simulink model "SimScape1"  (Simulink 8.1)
settings: Solver=ode45  StartTime=0.0  StopTime=.25  RelTol=1e-10
libraries: fl_lib x30, nesl_utility x6

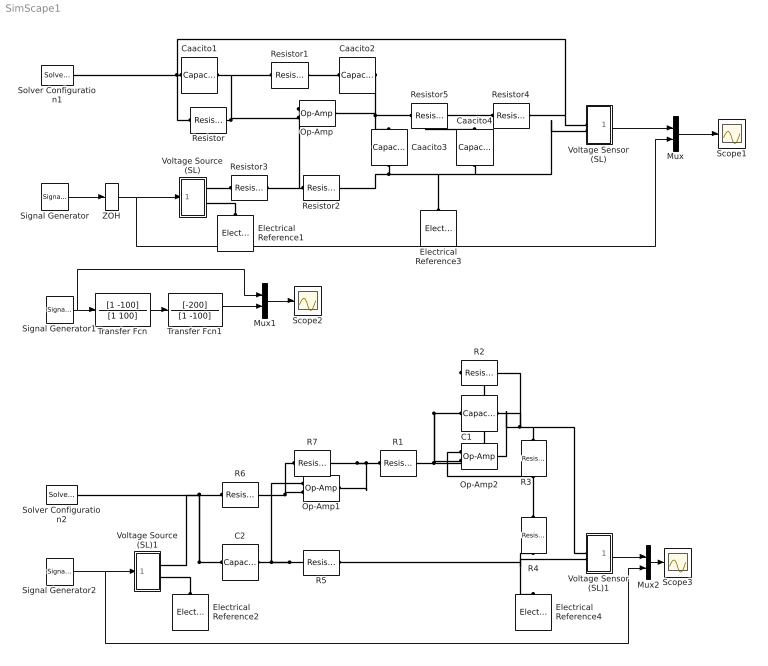
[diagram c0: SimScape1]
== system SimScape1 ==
  C1 : fl_lib/Electrical/Electrical Elements/Capacitor  c=2e-6 F  v0=0 V  r=1e-6 Ohm  g=0 1/Ohm  i_Log=off  v_Log=off  vc_Log=off  LocalVarNames=|i|v|vc  LocalVarDescs=|i|v|Internal variable for voltage across capacitor term  LocalVarLogging=[0 0 0]
  C2 : fl_lib/Electrical/Electrical Elements/Capacitor  c=1e-6 F  v0=0 V  r=1e-6 Ohm  g=0 1/Ohm  i_Log=off  v_Log=off  vc_Log=off  LocalVarNames=|i|v|vc  LocalVarDescs=|i|v|Internal variable for voltage across capacitor term  LocalVarLogging=[0 0 0]
  Caacito1 : fl_lib/Electrical/Electrical Elements/Capacitor  c=1e-6 F  v0=0 V  r=1e-6 Ohm  g=0 1/Ohm  i_Log=off  v_Log=off  vc_Log=off  LocalVarNames=|i|v|vc  LocalVarDescs=|i|v|Internal variable for voltage across capacitor term  LocalVarLogging=[0 0 0]
  Caacito2 : fl_lib/Electrical/Electrical Elements/Capacitor  c=1e-6 F  v0=0 V  r=1e-6 Ohm  g=0 1/Ohm  i_Log=off  v_Log=off  vc_Log=off  LocalVarNames=|i|v|vc  LocalVarDescs=|i|v|Internal variable for voltage across capacitor term  LocalVarLogging=[0 0 0]
  Caacito3 : fl_lib/Electrical/Electrical Elements/Capacitor  c=100e-6 F  v0=0 V  r=1e-6 Ohm  g=0 1/Ohm  i_Log=off  v_Log=off  vc_Log=off  LocalVarNames=|i|v|vc  LocalVarDescs=|i|v|Internal variable for voltage across capacitor term  LocalVarLogging=[0 0 0]
  Caacito4 : fl_lib/Electrical/Electrical Elements/Capacitor  c=100e-6 F  v0=0 V  r=1e-6 Ohm  g=0 1/Ohm  i_Log=off  v_Log=off  vc_Log=off  LocalVarNames=|i|v|vc  LocalVarDescs=|i|v|Internal variable for voltage across capacitor term  LocalVarLogging=[0 0 0]
  Electrical Reference{1..4} (4 alike) : fl_lib/Electrical/Electrical Elements/Electrical Reference  i_Log=off  LocalVarNames=|v1  LocalVarDescs=|v1  LocalVarLogging=[]
  Mux : Mux  Inputs=2
  Mux1 : Mux  Inputs=2
  Mux2 : Mux  Inputs=2
  Op-Amp : fl_lib/Electrical/Electrical Elements/Op-Amp  i1_Log=off  v1_Log=off  outI_Log=off  LocalVarNames=|i1|v1|outI  LocalVarDescs=|i1|v1|outI  LocalVarLogging=[0 0 0]
  Op-Amp1 : fl_lib/Electrical/Electrical Elements/Op-Amp  i1_Log=off  v1_Log=off  outI_Log=off  LocalVarNames=|i1|v1|outI  LocalVarDescs=|i1|v1|outI  LocalVarLogging=[0 0 0]
  Op-Amp2 : fl_lib/Electrical/Electrical Elements/Op-Amp  i1_Log=off  v1_Log=off  outI_Log=off  LocalVarNames=|i1|v1|outI  LocalVarDescs=|i1|v1|outI  LocalVarLogging=[0 0 0]
  R{1..3,5..7} (6 alike) : fl_lib/Electrical/Electrical Elements/Resistor  R=10 kOhm  i_Log=off  v_Log=off  LocalVarNames=|i|v  LocalVarDescs=|i|v  LocalVarLogging=[0 0]
  R4 : fl_lib/Electrical/Electrical Elements/Resistor  R=30 kOhm  i_Log=off  v_Log=off  LocalVarNames=|i|v  LocalVarDescs=|i|v  LocalVarLogging=[0 0]
  Resistor{,1..3} (4 alike) : fl_lib/Electrical/Electrical Elements/Resistor  R=1 kOhm  i_Log=off  v_Log=off  LocalVarNames=|i|v  LocalVarDescs=|i|v  LocalVarLogging=[0 0]
  Resistor4 : fl_lib/Electrical/Electrical Elements/Resistor  R=10 kOhm  i_Log=off  v_Log=off  LocalVarNames=|i|v  LocalVarDescs=|i|v  LocalVarLogging=[0 0]
  Resistor5 : fl_lib/Electrical/Electrical Elements/Resistor  R=10 kOhm  i_Log=off  v_Log=off  LocalVarNames=|i|v  LocalVarDescs=|i|v  LocalVarLogging=[0 0]
  Scope1 : Scope
  Scope2 : Scope
  Scope3 : Scope
  Signal Generator : SignalGenerator  WaveForm=square  Frequency=100
  Signal Generator1 : SignalGenerator  WaveForm=square  Frequency=10
  Signal Generator2 : SignalGenerator  WaveForm=square  Frequency=10
  Solver Configuration1 : nesl_utility/Solver Configuration  PhysicalDomain=network_engine_domain  SubClassName=solver  LeftPortType=input  RightPortType=generic  Accelerate=off  Tones=[]  Harmonics=[]  SimulateNoise=off  Profile=off  UseLocalSampling=off  EnableSwitchedLinearOptims=on  FrequencyDomain=off  UseCCode=off  UseNewInitialization=off  DoDC=off  ResidualTolerance=1e-4  UseLocalSolver=on  LocalSolverChoice=NE_BACKWARD_EULER_ADVANCER  LocalSolverSampleTime=.001  DoFixedCost=on  MaxNonlinIter=3  MaxModeIter=2  LinearAlgebra=Sparse  DelaysMemoryBudget=1024
  Solver Configuration2 : nesl_utility/Solver Configuration  PhysicalDomain=network_engine_domain  SubClassName=solver  LeftPortType=input  RightPortType=generic  Accelerate=off  Tones=[]  Harmonics=[]  SimulateNoise=off  Profile=off  UseLocalSampling=off  EnableSwitchedLinearOptims=on  FrequencyDomain=off  UseCCode=off  UseNewInitialization=off  DoDC=off  ResidualTolerance=1e-4  UseLocalSolver=on  LocalSolverChoice=NE_BACKWARD_EULER_ADVANCER  LocalSolverSampleTime=.001  DoFixedCost=on  MaxNonlinIter=3  MaxModeIter=2  LinearAlgebra=Sparse  DelaysMemoryBudget=1024
  Transfer Fcn : TransferFcn  Numerator=[1 -100]  Denominator=[1 100]
  Transfer Fcn1 : TransferFcn  Numerator=[-200]  Denominator=[1 -100]
  Voltage Sensor (SL) : Subsystem
  Voltage Sensor (SL)1 : Subsystem
  Voltage Source (SL) : Subsystem
  Voltage Source (SL)1 : Subsystem
  ZOH : ZeroOrderHold  SampleTime=.001
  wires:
  Signal Generator/1 -> ZOH/1
  Mux/1 -> Scope1/1
  Voltage Sensor (SL)/1(v) -> Mux/1
  ZOH/1 -> Voltage Source (SL)/1(S), Mux/2
  Signal Generator1/1 -> Transfer Fcn/1, Mux1/1
  Transfer Fcn/1 -> Transfer Fcn1/1
  Mux1/1 -> Scope2/1
  Transfer Fcn1/1 -> Mux1/2
  Signal Generator2/1 -> Voltage Source (SL)1/1(S), Mux2/2
  Mux2/1 -> Scope3/1
  Voltage Sensor (SL)1/1(v) -> Mux2/1
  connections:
  Caacito1/RConn1 -- Resistor/RConn1 -- Op-Amp/LConn2 -- Resistor1/LConn1
  Caacito1/LConn1 -- Resistor/LConn1 -- Resistor4/LConn1 -- Voltage Sensor (SL)/LConn1 -- Solver Configuration1/RConn1
  Resistor2/LConn1 -- Op-Amp/LConn1 -- Resistor3/LConn1
  Caacito2/LConn1 -- Resistor1/RConn1
  Caacito2/RConn1 -- Op-Amp/RConn1 -- Resistor5/RConn1 -- Caacito3/LConn1
  Resistor5/LConn1 -- Resistor4/RConn1 -- Caacito4/LConn1
  Caacito3/RConn1 -- Electrical Reference3/LConn1 -- Caacito4/RConn1 -- Voltage Sensor (SL)/LConn2 -- Resistor2/RConn1
  Electrical Reference1/LConn1 -- Voltage Source (SL)/RConn2
  Voltage Source (SL)/RConn1 -- Resistor3/RConn1
  R7/LConn1 -- R6/RConn1 -- Op-Amp1/LConn2
  C2/RConn1 -- Op-Amp1/LConn1 -- R5/LConn1
  R2/RConn1 -- C1/LConn1 -- Op-Amp2/LConn2 -- R1/RConn1
  R5/RConn1 -- R4/LConn1 -- Electrical Reference4/LConn1 -- Voltage Sensor (SL)1/LConn2
  Voltage Source (SL)1/RConn1 -- C2/LConn1 -- R6/LConn1 -- Solver Configuration2/RConn1
  Electrical Reference2/LConn1 -- Voltage Source (SL)1/RConn2
  R1/LConn1 -- R7/RConn1 -- Op-Amp1/RConn1
  R3/RConn1 -- C1/RConn1 -- Op-Amp2/RConn1 -- R2/LConn1 -- Voltage Sensor (SL)1/LConn1
  R3/LConn1 -- R4/RConn1 -- Op-Amp2/LConn1

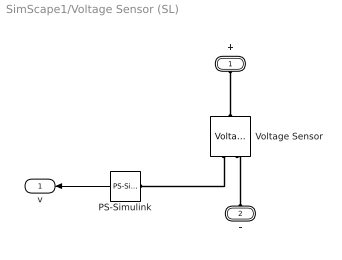
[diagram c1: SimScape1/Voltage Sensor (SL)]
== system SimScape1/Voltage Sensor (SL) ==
  PS-Simulink : nesl_utility/PS-Simulink Converter  PhysicalDomain=network_engine_domain  SubClassName=ps_output  LeftPortType=input  RightPortType=output  PseudoPeriodic=off  Frequencies=[]  Unit=V  AffineConversion=off
  Voltage Sensor : fl_lib/Electrical/Electrical Sensors/Voltage Sensor  i1_Log=off  v1_Log=off  LocalVarNames=|i1|v1  LocalVarDescs=|i1|v1  LocalVarLogging=[]
  + : PMIOPort  Port=1  Side=Left
  - : PMIOPort  Port=2  Side=Left
  v : Outport
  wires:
  PS-Simulink/1 -> v/1
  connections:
  Voltage Sensor/RConn1 -- PS-Simulink/LConn1
  +/RConn1 -- Voltage Sensor/LConn1
  -/RConn1 -- Voltage Sensor/RConn2

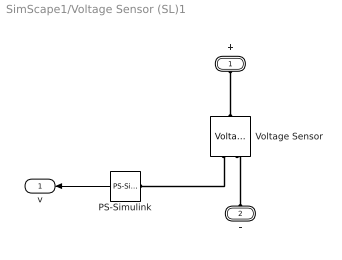
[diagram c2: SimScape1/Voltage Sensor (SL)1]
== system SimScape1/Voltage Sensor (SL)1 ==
  PS-Simulink : nesl_utility/PS-Simulink Converter  PhysicalDomain=network_engine_domain  SubClassName=ps_output  LeftPortType=input  RightPortType=output  PseudoPeriodic=off  Frequencies=[]  Unit=V  AffineConversion=off
  Voltage Sensor : fl_lib/Electrical/Electrical Sensors/Voltage Sensor  i1_Log=off  v1_Log=off  LocalVarNames=|i1|v1  LocalVarDescs=|i1|v1  LocalVarLogging=[]
  + : PMIOPort  Port=1  Side=Left
  - : PMIOPort  Port=2  Side=Left
  v : Outport
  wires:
  PS-Simulink/1 -> v/1
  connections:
  Voltage Sensor/RConn1 -- PS-Simulink/LConn1
  +/RConn1 -- Voltage Sensor/LConn1
  -/RConn1 -- Voltage Sensor/RConn2

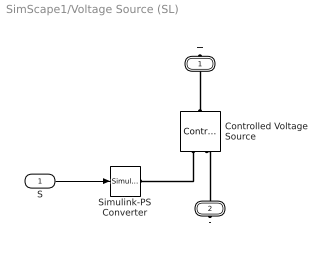
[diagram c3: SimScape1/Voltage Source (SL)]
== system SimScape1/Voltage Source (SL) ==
  S : Inport
  Controlled Voltage Source : fl_lib/Electrical/Electrical Sources/Controlled Voltage Source  i_Log=off  v_Log=off  LocalVarNames=|current|voltage|power  LocalVarDescs=|Current (A)|Voltage (V)|Power (W)  LocalVarLogging=[0 0 0]
  Simulink-PS Converter : nesl_utility/Simulink-PS Converter  PhysicalDomain=network_engine_domain  SubClassName=ps_input  LeftPortType=input  RightPortType=output  PseudoPeriodic=off  Frequencies=[]  NoiseDistribution=none  NoiseParameters=[]  Unit=V  AffineConversion=off  InputFiltering=off  SimscapeFilterOrder=1  InputFilterTimeConstant=.001  UdotUserProvided=0
  + : PMIOPort  Port=1  Side=Right
  - : PMIOPort  Port=2  Side=Right
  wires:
  S/1 -> Simulink-PS Converter/1
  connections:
  Controlled Voltage Source/RConn1 -- Simulink-PS Converter/RConn1
  -/RConn1 -- Controlled Voltage Source/RConn2
  +/RConn1 -- Controlled Voltage Source/LConn1

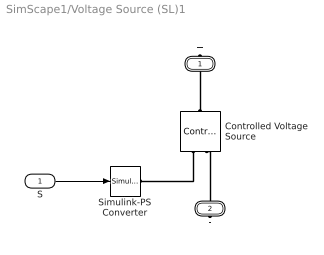
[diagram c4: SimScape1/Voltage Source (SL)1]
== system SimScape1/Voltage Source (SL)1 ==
  S : Inport
  Controlled Voltage Source : fl_lib/Electrical/Electrical Sources/Controlled Voltage Source  i_Log=off  v_Log=off  LocalVarNames=|current|voltage|power  LocalVarDescs=|Current (A)|Voltage (V)|Power (W)  LocalVarLogging=[0 0 0]
  Simulink-PS Converter : nesl_utility/Simulink-PS Converter  PhysicalDomain=network_engine_domain  SubClassName=ps_input  LeftPortType=input  RightPortType=output  PseudoPeriodic=off  Frequencies=[]  NoiseDistribution=none  NoiseParameters=[]  Unit=V  AffineConversion=off  InputFiltering=off  SimscapeFilterOrder=1  InputFilterTimeConstant=.001  UdotUserProvided=0
  + : PMIOPort  Port=1  Side=Right
  - : PMIOPort  Port=2  Side=Right
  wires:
  S/1 -> Simulink-PS Converter/1
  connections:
  Controlled Voltage Source/RConn1 -- Simulink-PS Converter/RConn1
  -/RConn1 -- Controlled Voltage Source/RConn2
  +/RConn1 -- Controlled Voltage Source/LConn1
